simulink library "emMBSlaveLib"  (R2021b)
settings: Solver=VariableStepAuto  StartTime=0.0  StopTime=10.0  RelTol=1e-3
undefined symbols (not defined in the file or in its folder): A, COM5

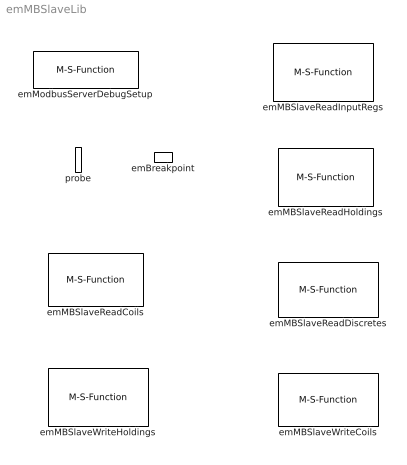
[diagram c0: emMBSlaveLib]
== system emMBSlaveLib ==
  emBreakpoint : M-S-Function  Tag=emBreakpoint  FunctionName=emBreakpoint2  Parameters=c_enableBK, c_times4break, c_continue,c_ObjID,c_serverID,c_UartNo,c_StartAddr4FirstBK,c_firstEnter  mask{c_enableBK=on, c_times4break=1, c_continue=off, c_ObjID=-1, c_serverID=0, c_UartNo=0, c_StartAddr4FirstBK=0, c_firstEnter=off}
      mask prompts: c_enableBK "Enable Breakpoint"; c_times4break "How many executing times to create one break ?"; c_continue "Continue Run (Now it is no use)"; c_ObjID "Obj_ID"; c_serverID "Debug Server ID"; c_UartNo "Debug Server uart"; c_StartAddr4FirstBK "Address of  First BK (0 based)"; c_firstEnter "First time enter this (change to exteral trigger by continur button)"
      mask init:
      | try
      | set_param(gcs,'Lock',"off");
      | set_param(gcbh,'MaskSelfModifiable',"on");
      | end
  emMBSlaveReadCoils : M-S-Function  FunctionName=emModbusSlaveReadCoils2  Parameters=c_ServerID,c_minAdr,c_RegQTY,c_sampleTime  mask(embedded Modbus Slave Read coils){c_ServerID=<empty>, c_minAdr=1, c_RegQTY=0, c_sampleTime=-1}
      mask prompts: c_ServerID "Modbus Server ID or node address:"; c_minAdr "MinAddress4Coil"; c_RegQTY "RegQTY4Coil"; c_sampleTime "Sample time in sec (-1 for inherited):"
      mask help: This is for embedded Modbus Server to update coil register values Input port "StartAddr" is coil register starting address ( 1 based without prefix 0X). Input port "Data" is scalar or vector which denotes coil register data source. It can be unconnected. When it is not connected, it means Data source is not from embedded target. The default size of Input port "Data" is 1 that is scalar. Data type of "Input port Data" must be boolean Output port "Data" is the same as Input port "Data" in both value and data type. Output port "Ok" true denotes all input data address range from this block is vali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
      mask init:
      | try
      |     set_param(gcs,'Lock',"off");
      |     set_param(gcbh,'MaskSelfModifiable',"on");
      | end
  emMBSlaveReadDiscretes : M-S-Function  FunctionName=emModbusSlaveReadDiscretes2  Parameters=c_ServerID,c_minAdr,c_RegQTY,c_sampleTime  mask(embedded Modbus Slave Read discrete inputs){c_ServerID=<empty>, c_minAdr=1, c_RegQTY=0, c_sampleTime=-1}
      mask prompts: c_ServerID "Modbus Server ID or node address:"; c_minAdr "MinAddress4Discrete"; c_RegQTY "RegQTY4Discrete"; c_sampleTime "Sample time in sec (-1 for inherited):"
      mask help: This is for embedded Modbus Server to update discrete register values Input port "StartAddr" is discrete register starting address ( 1 based without prefix 1X). Input port "Data" is scalar or vector which denotes discrete register data source. Data type of "Input port Data" must be boolean Output port "Data" is the same as Input port "Data" in both value and data type. Output port "Ok" true denotes all input data address range from this block is valid from Target firmware. And also true denotes communication OK between PC and Target from PC Debug/monitor software.
      mask init:
      | try
      |     set_param(gcs,'Lock',"off");
      |     set_param(gcbh,'MaskSelfModifiable',"on");
      | end
  emMBSlaveReadHoldings : M-S-Function  FunctionName=emModbusSlaveReadHolding2  Parameters=c_ServerID,c_OutputDataType,c_wordOrder,c_factor,c_minAdr,c_RegQTY,c_InPortDataType,c_sampleTime  mask(embedded Modbus Slave Read Holding registers){c_ServerID=<empty>, c_OutputDataType=uint32, c_wordOrder=big-endian, c_factor=1x, c_minAdr=0, c_RegQTY=0, c_InPortDataType=single, c_sampleTime=-1}
      mask prompts: c_ServerID "Modbus Server ID or node address:"; c_OutputDataType "Register data type:"; c_wordOrder "Word Order"; c_factor "Register Value  Factor for integer data type"; c_minAdr "MinAddress4Holding"; c_RegQTY "RegQTY4Holding"; c_InPortDataType "In Port "Data" type:"; c_sampleTime "Sample time in sec (-1 for inherited):"
      mask help: This is for embedded Modbus Server to update holding register values Input port "StartAddr" is holding register starting address ( 1 based without prefix 4X). Input port "Data" is scalar or vector which denotes holding register data source. It can be unconnected. When it is not connected, it means Data source is not from embedded target. The default size of Input port "Data" is 1 that is scalar. Data type of "Input port Data" can be "uint16, int16, uint32, int32, single" which is chosen by parameter. Data type of "holding register" can be different from Data type of "Input port Data" although 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
      mask init:
      | try
      |     set_param(gcs,'Lock',"off");
      |     set_param(gcbh,'MaskSelfModifiable',"on");
      | end
  emMBSlaveReadInputRegs : M-S-Function  FunctionName=emModbusSlaveReadInputRegs2  Parameters=c_ServerID,c_OutputDataType,c_wordOrder,c_factor,c_minAdr,c_RegQTY,c_InPortDataType,c_sampleTime  mask(embedded Modbus Slave Read Input registers){c_ServerID=<empty>, c_OutputDataType=uint16, c_wordOrder=big-endian, c_factor=1x, c_minAdr=1, c_RegQTY=0, c_InPortDataType=uint16, c_sampleTime=-1}
      mask prompts: c_ServerID "Modbus Server ID or node address:"; c_OutputDataType "Register data type:"; c_wordOrder "Word Order"; c_factor "Value  Factor for integer data type when reg and In port "Data" have different type"; c_minAdr "MinAddress4InputReg"; c_RegQTY "RegQTY4InputReg"; c_InPortDataType "In-Port "Data" type:"; c_sampleTime "Sample time in sec (-1 for inherited):"
      mask help: This is for embedded Modbus Server to update input register values Input port "StartAddr" is Input register starting address ( 1 based without prefix 3X). Input port "Data" is scalar or vector which denotes input register data source. Data type of "Input port Data" can be "uint16, int16, uint32, int32, single" which is chosen by parameter. Data type of "input register" can be different from Data type of "Input port Data" although Data type of "input register" can be "uint16, int16, uint32, int32, single". When data type of "Input port Data" is "single" and data type of "input register" is "uin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
      mask init:
      | try
      |     set_param(gcs,'Lock',"off");
      |     set_param(gcbh,'MaskSelfModifiable',"on");
      | end
  emMBSlaveWriteCoils : M-S-Function  FunctionName=emModbusSlaveWriteCoils2  Parameters=c_ServerID,c_UartNo,c_minAdr,c_RegQTY,c_singleWriting,c_sampleTime  mask(embedded Modbus Slave Write Coils){c_ServerID=<empty>, c_UartNo=1, c_minAdr=1, c_RegQTY=1, c_singleWriting=off, c_sampleTime=-1}
      mask prompts: c_ServerID "Modbus Server ID or node address:"; c_UartNo "Uart No (In case 2 or 2+ Uarts with the same Server ID)"; c_minAdr "MinAddress4Coil"; c_RegQTY "RegQTY4Coil"; c_singleWriting "Use Single Coil Reg writing"; c_sampleTime "Sample time in sec (-1 for inherited):"
      mask help: This is for writing coil registers. How many items will be written? The written item Qty value is Input port "Data" vector size. Coli reg Value is equal to Input Port "Data". Input port "StartAddr" provides 1-based start address without 0x prefix (uint16 type)., which is from embedded target. PC can use probe to monitor if it is not constant. Input Port "Data" is allowed to connect constant vector block in embedded target model. The embedded target only uses size of input port "Data" vector information for embedded target code. If Input Port "Data" is unconnected, the default size is 1. Input 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
      mask init:
      | try
      |     set_param(gcs,'Lock',"off");
      |     set_param(gcbh,'MaskSelfModifiable',"on");
      | end
  emMBSlaveWriteHoldings : M-S-Function  FunctionName=emModbusSlaveWriteHoldings2  Parameters=c_ServerID,c_UartNo,c_OutputDataType,c_wordOrder,c_factor,c_minAdr,c_RegQTY,c_singleWriting,c_DataPortType,c_sampleTime  mask(embedded Modbus Slave Writie holdings){c_ServerID=<empty>, c_UartNo=2, c_OutputDataType=uint16, c_wordOrder=big-endian, c_factor=1x, c_minAdr=1, c_RegQTY=65, c_singleWriting=off, c_DataPortType=single, c_sampleTime=-1}
      mask prompts: c_ServerID "Modbus Server ID or node address:"; c_UartNo "Uart No (In case 2 or 2+ Uarts with the same Server ID)"; c_OutputDataType "Holding Register data type:"; c_wordOrder "Word Order"; c_factor "Value  Factor for integer data type when reg and out port "Data" have different type"; c_minAdr "MinAddress4Holding"; c_RegQTY "RegQTY4Holding"; c_singleWriting "Use Single holding Reg writing"; c_DataPortType "Out port "Data" type"; c_sampleTime "Sample time in sec (-1 for inherited):"
      mask help: This is for embedded target to get holding registers value which is written by PC or external Modbus client . How many items will be written? The written item unit is paramter "register data type". The written item Qty value is Input port "Data" vector size. Holding reg Value is equal to Input Port "Data" when Holding reg type is "single". Holding reg Value is equal to Input Port "Data" x Factor when Holding reg type is "uint16/int16/uint32/int32" and outport data type is single. Input port "StartAddr" provides 1-based start address without 4x prefix (uint16 type), which is from embedded targe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
      mask init:
      | try
      |     set_param(gcs,'Lock',"off");
      |     set_param(gcbh,'MaskSelfModifiable',"on");
      | end
  emModbusServerDebugSetup : M-S-Function  Tag=emModbusSlaveSetup  FunctionName=emModbusSlaveDebugSetup2  Parameters=c_objID,c_uartNo,c_baudrate,c_serverID,c_baudrate4PC,c_forceLongerSpace,c_holdingRegsQTY,c_minHoldingAddr,c_inputRegsQTY,c_minInputRegAddr,c_coilRegsQTY,c_minCoilAddr,c_discreteRegsQTY,c_minDiscreteAddr,c_enableDebug,c_emWaitQTY,c_breakpointMaxQTY,c_probeMaxWordQTY,g_COMPortNo,c_Name_method,c_PortName,c_BitNo,c_TxEnable485,c_TxEnable485Polarity  mask(embedded Modbus Server/Debug setup){c_objID=0, c_uartNo=4, c_baudrate=19200, c_serverID=1, c_baudrate4PC=115200, c_forceLongerSpace=on, c_holdingRegsQTY=65000, c_minHoldingAddr=789, c_inputRegsQTY=200, c_minInputRegAddr=20, c_coilRegsQTY=300, c_minCoilAddr=30, c_discreteRegsQTY=400, c_minDiscreteAddr=40, c_enableDebug=on, c_breakpointMaxQTY=100, c_probeMaxWordQTY=200, c_emWaitQTY=0, g_COMPortNo=COM5, c_Name_method=By C language writing variable/macro name, c_PortName=A, c_BitNo=1, c_TxEnable485="LATAbits.LATA1", c_TxEnable485Polarity=on}
      mask prompts: c_objID "Object ID for multiple Modbus salve/debug Hardware"; c_uartNo "embedded target UART No:"; c_baudrate "embedded target Baud Rate:"; c_serverID "embedded target modbus server ID:"; c_baudrate4PC "PC Side USB/Bluetooth Serial Port Baud Rate"; c_forceLongerSpace "Force longer space"; c_holdingRegsQTY "Holding Regs Qty:"; c_minHoldingAddr "Min Holding Reg address (1-based without 4x prefix):"; c_inputRegsQTY "Input Regs Qty:"; c_minInputRegAddr "Min Input Reg address (1-based without 3x prefix):"; c_coilRegsQTY "Coil Regs Qty:"; c_minCoilAddr "Min Coil Reg address (1-based without 0x prefix):"; c_discreteRegsQTY "Discrete Regs Qty:"; c_minDiscreteAddr "Min Discrete Reg address (1-based without 1x prefix):"; c_enableDebug "Enable Debug/Monitor by this hardware"; c_breakpointMaxQTY "Break points MAX Qty:"; c_probeMaxWordQTY "Max words QTY by all Probe variables use:"; c_emWaitQTY "Max Qty for embedded wait block (emWait):"; g_COMPortNo "PC Com Port for Debug or Monitor:"; c_Name_method "How to specify Tx Enable Port:"; c_PortName "Port Name:"; c_BitNo "Port Bit number::"; c_TxEnable485 "RS485 Tx En C Name:"; c_TxEnable485Polarity "Target RS485 Tx Enable polarity is High"
      mask help: This block will setup embedded Modbus or Debug/Monitor all parameters
      mask init:
      | try
      |     set_param(gcs,'Lock',"off");
      |     set_param(gcbh,'MaskSelfModifiable',"on");
      | end
  probe : M-S-Function  Tag=emProbe  FunctionName=emProbe2  Parameters=c_ObjID,c_serverID,c_UartNo,c_StartAddr,c_ConstantDataSource  mask(embedded Probe){c_ObjID=-1, c_serverID=1, c_UartNo=4, c_StartAddr=[], c_ConstantDataSource=on}
      mask prompts: c_ObjID "Obj_ID"; c_serverID "Debug Server ID"; c_UartNo "Debug Server uart"; c_StartAddr "Address of  Mine (1 based)"; c_ConstantDataSource "Constant Source Data"
      mask help: Probe is used for watching Simulink Signal by connecting "Display" block
      mask init:
      | try
      |     set_param(gcs,'Lock',"off");
      |     set_param(gcbh,'MaskSelfModifiable',"on");
      | end
